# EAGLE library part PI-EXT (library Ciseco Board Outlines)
Ciseco Rasbperry Pi add on board outlines This version includes two headers joined together
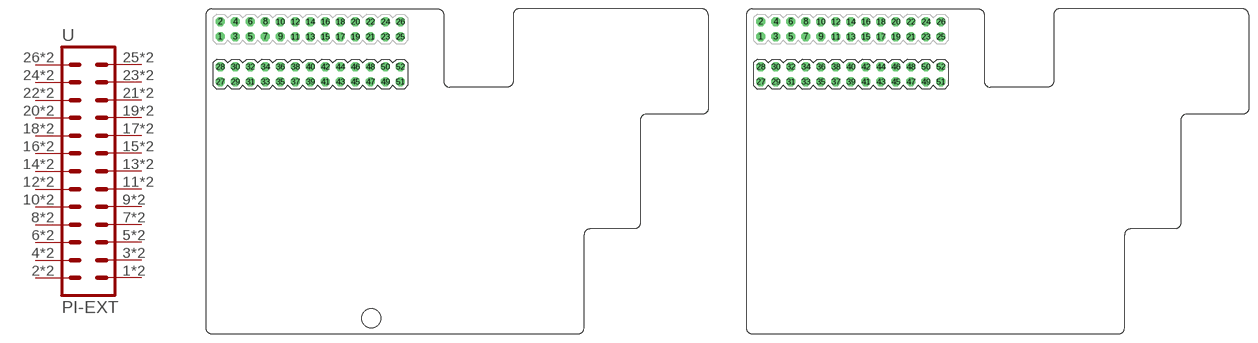
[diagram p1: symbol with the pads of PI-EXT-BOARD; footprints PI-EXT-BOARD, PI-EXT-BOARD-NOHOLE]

Designator prefix U

## PI-EXT-BOARD  [PI-EXT-BOARD]
1  1  pas
2  2  pas
3  3  pas
4  4  pas
5  5  pas
6  6  pas
7  7  pas
8  8  pas
9  9  pas
10  10  pas
11  11  pas
12  12  pas
13  13  pas
14  14  pas
15  15  pas
16  16  pas
17  17  pas
18  18  pas
19  19  pas
20  20  pas
21  21  pas
22  22  pas
23  23  pas
24  24  pas
25  25  pas
26  26  pas
27  1  pas
28  2  pas
29  3  pas
30  4  pas
31  5  pas
32  6  pas
33  7  pas
34  8  pas
35  9  pas
36  10  pas
37  11  pas
38  12  pas
39  13  pas
40  14  pas
41  15  pas
42  16  pas
43  17  pas
44  18  pas
45  19  pas
46  20  pas
47  21  pas
48  22  pas
49  23  pas
50  24  pas
51  25  pas
52  26  pas

## PI-EXT-BOARD-NOHOLE  [PI-EXT-BOARD-NOHOLE]
Pads as for PI-EXT-BOARD

## PI-EXT-BOARD-REF  [PI-EXT-BOARD-REF]
Pads as for PI-EXT-BOARD

## PI-EXT-BOARD-PI-LITE  [PI-LITE-EXT-BOARD]
Pads as for PI-EXT-BOARD

## Footprint PI-EXT-BOARD (pad centres in mm)
drill 1.016 octagon: 1 2.44,50.31; 2 2.44,52.85; 3 4.98,50.31; 4 4.98,52.85; 5 7.52,50.31; 6 7.52,52.85; 7 10.06,50.31; 8 10.06,52.85; 9 12.6,50.31; 10 12.6,52.85; 11 15.14,50.31; 12 15.14,52.85; 13 17.68,50.31; 14 17.68,52.85; 15 20.22,50.31; 16 20.22,52.85; 17 22.76,50.31; 18 22.76,52.85; 19 25.3,50.31; 20 25.3,52.85; 21 27.84,50.31; 22 27.84,52.85; 23 30.38,50.31; 24 30.38,52.85; 25 32.92,50.31; 26 32.92,52.85; 27 2.44,42.69; 28 2.44,45.23; 29 4.98,42.69; 30 4.98,45.23; 31 7.52,42.69; 32 7.52,45.23; 33 10.06,42.69; 34 10.06,45.23; 35 12.6,42.69; 36 12.6,45.23; 37 15.14,42.69; 38 15.14,45.23; 39 17.68,42.69; 40 17.68,45.23; 41 20.22,42.69; 42 20.22,45.23; 43 22.76,42.69; 44 22.76,45.23; 45 25.3,42.69; 46 25.3,45.23; 47 27.84,42.69; 48 27.84,45.23; 49 30.38,42.69; 50 30.38,45.23; 51 32.92,42.69; 52 32.92,45.23
hole 3.2 at 28.019,2.638

## Footprint PI-EXT-BOARD-NOHOLE (pad centres in mm)
drill 1.016 octagon: 1 2.44,50.31; 2 2.44,52.85; 3 4.98,50.31; 4 4.98,52.85; 5 7.52,50.31; 6 7.52,52.85; 7 10.06,50.31; 8 10.06,52.85; 9 12.6,50.31; 10 12.6,52.85; 11 15.14,50.31; 12 15.14,52.85; 13 17.68,50.31; 14 17.68,52.85; 15 20.22,50.31; 16 20.22,52.85; 17 22.76,50.31; 18 22.76,52.85; 19 25.3,50.31; 20 25.3,52.85; 21 27.84,50.31; 22 27.84,52.85; 23 30.38,50.31; 24 30.38,52.85; 25 32.92,50.31; 26 32.92,52.85; 27 2.44,42.69; 28 2.44,45.23; 29 4.98,42.69; 30 4.98,45.23; 31 7.52,42.69; 32 7.52,45.23; 33 10.06,42.69; 34 10.06,45.23; 35 12.6,42.69; 36 12.6,45.23; 37 15.14,42.69; 38 15.14,45.23; 39 17.68,42.69; 40 17.68,45.23; 41 20.22,42.69; 42 20.22,45.23; 43 22.76,42.69; 44 22.76,45.23; 45 25.3,42.69; 46 25.3,45.23; 47 27.84,42.69; 48 27.84,45.23; 49 30.38,42.69; 50 30.38,45.23; 51 32.92,42.69; 52 32.92,45.23

## Footprint PI-EXT-BOARD-REF (pad centres in mm)
drill 1.016 octagon: 1 2.44,50.31; 2 2.44,52.85; 3 4.98,50.31; 4 4.98,52.85; 5 7.52,50.31; 6 7.52,52.85; 7 10.06,50.31; 8 10.06,52.85; 9 12.6,50.31; 10 12.6,52.85; 11 15.14,50.31; 12 15.14,52.85; 13 17.68,50.31; 14 17.68,52.85; 15 20.22,50.31; 16 20.22,52.85; 17 22.76,50.31; 18 22.76,52.85; 19 25.3,50.31; 20 25.3,52.85; 21 27.84,50.31; 22 27.84,52.85; 23 30.38,50.31; 24 30.38,52.85; 25 32.92,50.31; 26 32.92,52.85; 27 2.44,42.69; 28 2.44,45.23; 29 4.98,42.69; 30 4.98,45.23; 31 7.52,42.69; 32 7.52,45.23; 33 10.06,42.69; 34 10.06,45.23; 35 12.6,42.69; 36 12.6,45.23; 37 15.14,42.69; 38 15.14,45.23; 39 17.68,42.69; 40 17.68,45.23; 41 20.22,42.69; 42 20.22,45.23; 43 22.76,42.69; 44 22.76,45.23; 45 25.3,42.69; 46 25.3,45.23; 47 27.84,42.69; 48 27.84,45.23; 49 30.38,42.69; 50 30.38,45.23; 51 32.92,42.69; 52 32.92,45.23

## Footprint PI-LITE-EXT-BOARD (pad centres in mm)
drill 1.016 octagon: 1 2.44,50.31; 2 2.44,52.85; 3 4.98,50.31; 4 4.98,52.85; 5 7.52,50.31; 6 7.52,52.85; 7 10.06,50.31; 8 10.06,52.85; 9 12.6,50.31; 10 12.6,52.85; 11 15.14,50.31; 12 15.14,52.85; 13 17.68,50.31; 14 17.68,52.85; 15 20.22,50.31; 16 20.22,52.85; 17 22.76,50.31; 18 22.76,52.85; 19 25.3,50.31; 20 25.3,52.85; 21 27.84,50.31; 22 27.84,52.85; 23 30.38,50.31; 24 30.38,52.85; 25 32.92,50.31; 26 32.92,52.85; 27 2.44,42.69; 28 2.44,45.23; 29 4.98,42.69; 30 4.98,45.23; 31 7.52,42.69; 32 7.52,45.23; 33 10.06,42.69; 34 10.06,45.23; 35 12.6,42.69; 36 12.6,45.23; 37 15.14,42.69; 38 15.14,45.23; 39 17.68,42.69; 40 17.68,45.23; 41 20.22,42.69; 42 20.22,45.23; 43 22.76,42.69; 44 22.76,45.23; 45 25.3,42.69; 46 25.3,45.23; 47 27.84,42.69; 48 27.84,45.23; 49 30.38,42.69; 50 30.38,45.23; 51 32.92,42.69; 52 32.92,45.23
